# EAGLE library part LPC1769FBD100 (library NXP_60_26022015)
32-bit ARM Cortex-M3 microcontroller; up to 512 kB flash and 64 kB SRAM with Ethernet, USB 2.0 Host/Device/OTG, CAN The LPC1769/68/67/66/65/64/63 are ARM Cortex-M3 based microcontrollers for embedded applications featuring a high level of integration and low power consumption. The ARM Cortex-M3 is a next generation core that offers system enhancements such as enhanced debug features and a higher level of support block integration. The LPC1768/67/66/65/64/63 operate at CPU frequencies of up to 100 MHz. The LPC1769 operates at CPU frequencies of up to 120 MHz. The ARM Cortex-M3 CPU incorporates a 3-stage pipeline and uses a Harvard architecture with separate local instruction and data buses as well as a third bus for peripherals. The ARM Cortex-M3 CPU also includes an internal prefetch unit that supports speculative branching. The peripheral complement of the LPC1769/68/67/66/65/64/63 includes up to 512 kB of flash memory, up to 64 kB of data memory, Ethernet MAC, USB Device/Host/OTG interface, 8-channel general purpose DMA controller, 4 UARTs, 2 CAN channels, 2 SSP controllers, SPI interface, 3 I 2 C-bus interfaces, 2-input plus 2-output I 2 S-bus interface, 8-channel 12-bit ADC, 10-bit DAC, motor control PWM, Quadrature Encoder interface, four general purpose timers, 6-output general purpose PWM, ultra-low power Real-Time Clock (RTC) with separate battery supply, and up to 70 general purpose I/O pins. The LPC1769/68/67/66/65/64/63 are pin-compatible to the 100-pin LPC236x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
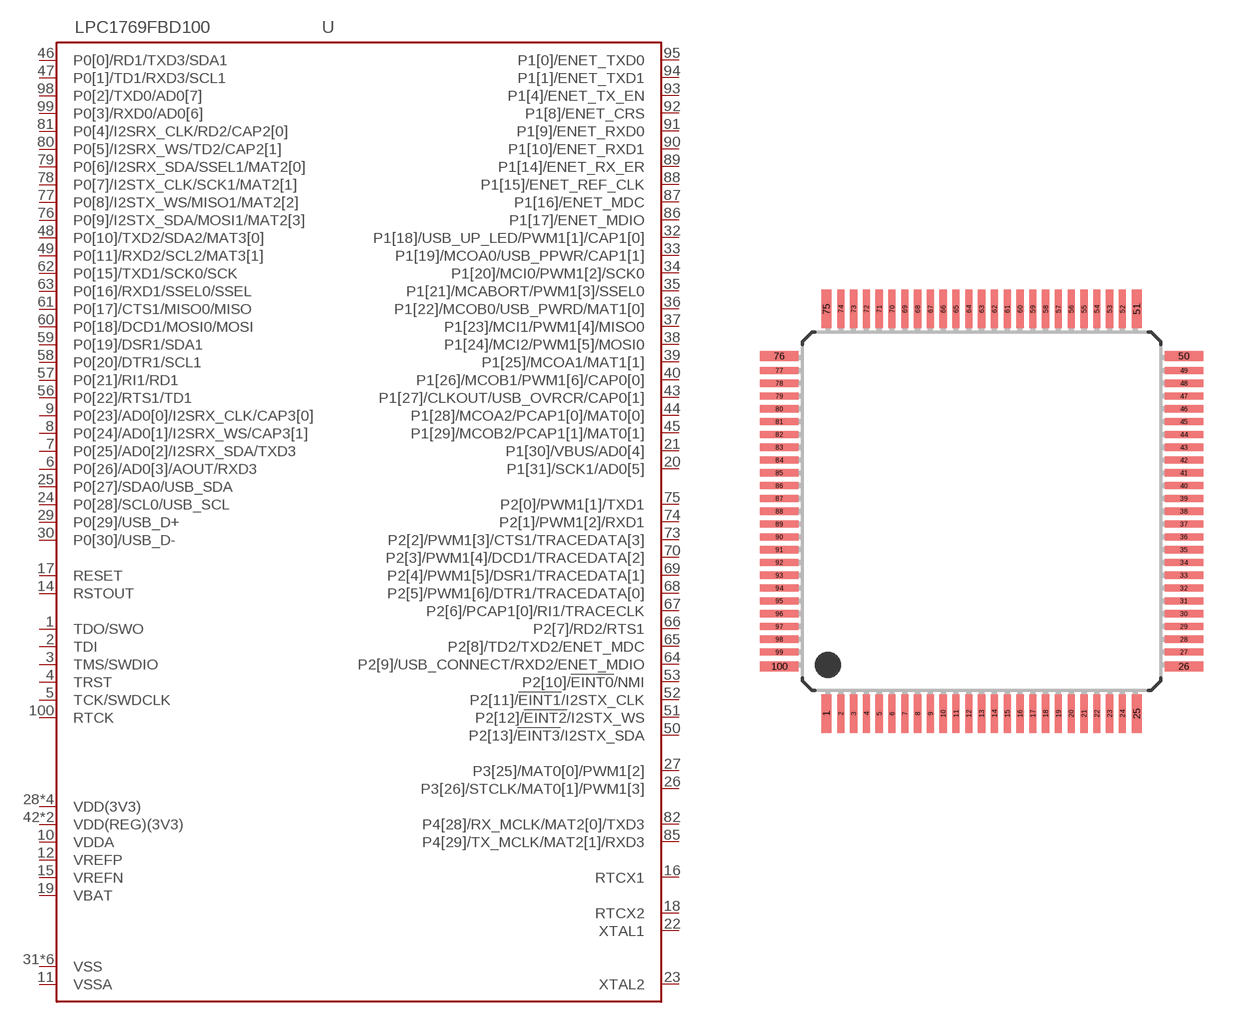
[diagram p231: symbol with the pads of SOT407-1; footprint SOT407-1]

Designator prefix U

## LPC1769FBD100 (CAN: yes; DAC: yes; ETH: yes; FLASH: 512kB; I2S: yes; MHZ: 120; SRAM: 32kB; SRAM0: 16kB; SRAM1: 16kB; USB: D/H/OTG)  [SOT407-1]
1  TDO/SWO
2  TDI
3  TMS/SWDIO
4  TRST
5  TCK/SWDCLK
6  P0[26]/AD0[3]/AOUT/RXD3
7  P0[25]/AD0[2]/I2SRX_SDA/TXD3
8  P0[24]/AD0[1]/I2SRX_WS/CAP3[1]
9  P0[23]/AD0[0]/I2SRX_CLK/CAP3[0]
10  VDDA
11  VSSA
12  VREFP
14  RSTOUT
15  VREFN
16  RTCX1
17  RESET
18  RTCX2
19  VBAT
20  P1[31]/SCK1/AD0[5]
21  P1[30]/VBUS/AD0[4]
22  XTAL1
23  XTAL2
24  P0[28]/SCL0/USB_SCL
25  P0[27]/SDA0/USB_SDA
26  P3[26]/STCLK/MAT0[1]/PWM1[3]
27  P3[25]/MAT0[0]/PWM1[2]
28  VDD(3V3)
29  P0[29]/USB_D+
30  P0[30]/USB_D-
31  VSS
32  P1[18]/USB_UP_LED/PWM1[1]/CAP1[0]
33  P1[19]/MCOA0/USB_PPWR/CAP1[1]
34  P1[20]/MCI0/PWM1[2]/SCK0
35  P1[21]/MCABORT/PWM1[3]/SSEL0
36  P1[22]/MCOB0/USB_PWRD/MAT1[0]
37  P1[23]/MCI1/PWM1[4]/MISO0
38  P1[24]/MCI2/PWM1[5]/MOSI0
39  P1[25]/MCOA1/MAT1[1]
40  P1[26]/MCOB1/PWM1[6]/CAP0[0]
41  VSS
42  VDD(REG)(3V3)
43  P1[27]/CLKOUT/USB_OVRCR/CAP0[1]
44  P1[28]/MCOA2/PCAP1[0]/MAT0[0]
45  P1[29]/MCOB2/PCAP1[1]/MAT0[1]
46  P0[0]/RD1/TXD3/SDA1
47  P0[1]/TD1/RXD3/SCL1
48  P0[10]/TXD2/SDA2/MAT3[0]
49  P0[11]/RXD2/SCL2/MAT3[1]
50  P2[13]/!EINT3!/I2STX_SDA
51  P2[12]/!EINT2!/I2STX_WS
52  P2[11]/!EINT1!/I2STX_CLK
53  P2[10]/!EINT0!/NMI
54  VDD(3V3)
55  VSS
56  P0[22]/RTS1/TD1
57  P0[21]/RI1/RD1
58  P0[20]/DTR1/SCL1
59  P0[19]/DSR1/SDA1
60  P0[18]/DCD1/MOSI0/MOSI
61  P0[17]/CTS1/MISO0/MISO
62  P0[15]/TXD1/SCK0/SCK
63  P0[16]/RXD1/SSEL0/SSEL
64  P2[9]/USB_CONNECT/RXD2/ENET_MDIO
65  P2[8]/TD2/TXD2/ENET_MDC
66  P2[7]/RD2/RTS1
67  P2[6]/PCAP1[0]/RI1/TRACECLK
68  P2[5]/PWM1[6]/DTR1/TRACEDATA[0]
69  P2[4]/PWM1[5]/DSR1/TRACEDATA[1]
70  P2[3]/PWM1[4]/DCD1/TRACEDATA[2]
71  VDD(3V3)
72  VSS
73  P2[2]/PWM1[3]/CTS1/TRACEDATA[3]
74  P2[1]/PWM1[2]/RXD1
75  P2[0]/PWM1[1]/TXD1
76  P0[9]/I2STX_SDA/MOSI1/MAT2[3]
77  P0[8]/I2STX_WS/MISO1/MAT2[2]
78  P0[7]/I2STX_CLK/SCK1/MAT2[1]
79  P0[6]/I2SRX_SDA/SSEL1/MAT2[0]
80  P0[5]/I2SRX_WS/TD2/CAP2[1]
81  P0[4]/I2SRX_CLK/RD2/CAP2[0]
82  P4[28]/RX_MCLK/MAT2[0]/TXD3
83  VSS
84  VDD(REG)(3V3)
85  P4[29]/TX_MCLK/MAT2[1]/RXD3
86  P1[17]/ENET_MDIO
87  P1[16]/ENET_MDC
88  P1[15]/ENET_REF_CLK
89  P1[14]/ENET_RX_ER
90  P1[10]/ENET_RXD1
91  P1[9]/ENET_RXD0
92  P1[8]/ENET_CRS
93  P1[4]/ENET_TX_EN
94  P1[1]/ENET_TXD1
95  P1[0]/ENET_TXD0
96  VDD(3V3)
97  VSS
98  P0[2]/TXD0/AD0[7]
99  P0[3]/RXD0/AD0[6]
100  RTCK

## Footprint SOT407-1 (pad centres in mm)
SOT407-1 LQFP100: plastic low profile quad flat package; 100 leads; body 14 x 14 x 1.4 mm JEDEC: MS-026 IEC: 136E20
smd 0.4 x 1.5: 1 -6.06,-7.9; 25 6.06,-7.9; 51 6.06,7.9; 75 -6.06,7.9
smd 0.28 x 1.5: 2 -5.5,-7.9; 3 -5,-7.9; 4 -4.5,-7.9; 5 -4,-7.9; 6 -3.5,-7.9; 7 -3,-7.9; 8 -2.5,-7.9; 9 -2,-7.9; 10 -1.5,-7.9; 11 -1,-7.9; 12 -0.5,-7.9; 13 0,-7.9; 14 0.5,-7.9; 15 1,-7.9; 16 1.5,-7.9; 17 2,-7.9; 18 2.5,-7.9; 19 3,-7.9; 20 3.5,-7.9; 21 4,-7.9; 22 4.5,-7.9; 23 5,-7.9; 24 5.5,-7.9; 52 5.5,7.9; 53 5,7.9; 54 4.5,7.9; 55 4,7.9; 56 3.5,7.9; 57 3,7.9; 58 2.5,7.9; 59 2,7.9; 60 1.5,7.9; 61 1,7.9; 62 0.5,7.9; 63 0,7.9; 64 -0.5,7.9; 65 -1,7.9; 66 -1.5,7.9; 67 -2,7.9; 68 -2.5,7.9; 69 -3,7.9; 70 -3.5,7.9; 71 -4,7.9; 72 -4.5,7.9; 73 -5,7.9; 74 -5.5,7.9
smd 1.5 x 0.4: 26 7.9,-6.06; 50 7.9,6.06; 76 -7.9,6.06; 100 -7.9,-6.06
smd 1.5 x 0.28: 27 7.9,-5.5; 28 7.9,-5; 29 7.9,-4.5; 30 7.9,-4; 31 7.9,-3.5; 32 7.9,-3; 33 7.9,-2.5; 34 7.9,-2; 35 7.9,-1.5; 36 7.9,-1; 37 7.9,-0.5; 38 7.9,0; 39 7.9,0.5; 40 7.9,1; 41 7.9,1.5; 42 7.9,2; 43 7.9,2.5; 44 7.9,3; 45 7.9,3.5; 46 7.9,4; 47 7.9,4.5; 48 7.9,5; 49 7.9,5.5; 77 -7.9,5.5; 78 -7.9,5; 79 -7.9,4.5; 80 -7.9,4; 81 -7.9,3.5; 82 -7.9,3; 83 -7.9,2.5; 84 -7.9,2; 85 -7.9,1.5; 86 -7.9,1; 87 -7.9,0.5; 88 -7.9,0; 89 -7.9,-0.5; 90 -7.9,-1; 91 -7.9,-1.5; 92 -7.9,-2; 93 -7.9,-2.5; 94 -7.9,-3; 95 -7.9,-3.5; 96 -7.9,-4; 97 -7.9,-4.5; 98 -7.9,-5; 99 -7.9,-5.5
